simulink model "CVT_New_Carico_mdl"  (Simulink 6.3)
settings: Solver=ode15s  StartTime=0.0  StopTime=10.0  RelTol=1e-8  AbsTol=1e-8
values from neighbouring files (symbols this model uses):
  b_0 = kb*J_0    (= 0.00382059739779)    [CVT_New.m]    (also in CVT_New_th.m)
  b_mn = b_m+b_n*(Nm/Nn1)^2    (= 0.0609042388033)    [CVT_New.m]    (also in CVT_New_th.m)
  b_op = b_p+b_o*(Np/No)^2    (= 0.00942365042771)    [CVT_New.m]    (also in CVT_New_th.m)
  b_qt = b_q+b_t*(Nq/Nt1)^2    (= 0.0289383393218)    [CVT_New.m]    (also in CVT_New_th.m)
  b_r = kb*J_r    (= 218.026030555)    [architetture_epicicloidale_statico.m]    (also in architetture_HEV_startstop_1.m = 21.8026030555; architetture_HEV_startstop_2.m = 21.8026030555; CVT_New.m = 0.218026030555; CVT_New_th.m = 0.218026030555)
  Bs0 = diag([b_s,b_s0])    [CVT_New.m]    (also in CVT_New_th.m)
  C_pq = 1e-14*m^3/Pa    (= 1e-14)    [CVT_New.m]    (also in CVT_New_th.m)
  d_0s = d0    (= 10)    [CVT_New.m]    (also in CVT_New_th.m)
  d_m0 = d0    (= 10)    [CVT_New.m]    (also in CVT_New_th.m)
  d_pm = d0    (= 10)    [CVT_New.m]    (also in CVT_New_th.m)
  d_qr = d0    (= 10)    [CVT_New.m]    (also in CVT_New_th.m)
  d_sr = d0    (= 10)    [CVT_New.m]    (also in CVT_New_th.m; architetture_epicicloidale.m; architetture_epicicloidale_cont.m; architetture_epicicloidale_prova.m)
  Hp_max = Hq    (= 1.8724110952e-05)    [CVT_New.m]    (also in CVT_New_th.m)
  Hq = (400*lt/minuti)/(3400*rpm)    (= 1.8724110952e-05)    [CVT_New.m]    (also in CVT_New_th.m)
  J_0 = 1.3*0.5*pi*rho_acc*h0*r_0^4    (= 3.82059739779e-05)    [CVT_New.m]    (also in CVT_New_th.m)
  J_mn = J_m+J_n*(Nm/Nn1)^2    (= 0.000609042388033)    [CVT_New.m]    (also in CVT_New_th.m)
  J_op = J_p+J_o*(Np/No)^2    (= 9.42365042771e-05)    [CVT_New.m]    (also in CVT_New_th.m)
  J_qt = J_q+J_t*(Nq/Nt1)^2    (= 0.000289383393218)    [CVT_New.m]    (also in CVT_New_th.m)
  J_r = 0.5*pi*rho_acc*(hr*r_r^4 + h_ring*(r_re^4-r_r^4))    (= 2.18026030555)    [architetture_epicicloidale_statico.m]    (also in architetture_HEV_startstop_1.m; architetture_HEV_startstop_2.m; CVT_New.m = 0.00218026030555; CVT_New_th.m = 0.00218026030555)
  JJs0 = diag([J_s,J_s0])    [CVT_New.m]    (also in CVT_New_th.m)
  K_0s = K0    (= 1000000)    [CVT_New.m]    (also in CVT_New_th.m)
  K_m0 = K0    (= 1000000)    [CVT_New.m]    (also in CVT_New_th.m)
  K_pm = K0    (= 1000000)    [CVT_New.m]    (also in CVT_New_th.m)
  K_qr = K0    (= 1000000)    [CVT_New.m]    (also in CVT_New_th.m)
  K_sr = K0    (= 1000000)    [CVT_New.m]    (also in CVT_New_th.m; architetture_epicicloidale.m = 10000000; architetture_epicicloidale_cont.m = 10000000; architetture_epicicloidale_prova.m = 10000000)
  Mv = 4000*kg    (= 4000)    [CVT_New.m]    (also in CVT_New_th.m)
  Ppq_0 = 0    [CVT_New.m]    (also in CVT_New_th.m)
  r_0 = xd0*N0/(2*pi)    (= 0.0954929658551)    [CVT_New.m]    (also in CVT_New_th.m)
  r_mn = (Nm/Nn1)*r_n2    (= 0.148158783387)    [CVT_New.m]    (also in CVT_New_th.m)
  r_op = (Np/No)*r_o    (= 0.105042262441)    [CVT_New.m]    (also in CVT_New_th.m)
  R_p = 0.8*(30*bar)/(400*lt/minuti)    (= 360000000)    [CVT_New.m]    (also in CVT_New_th.m)
  R_q = 0.8*(30*bar)/(400*lt/minuti)    (= 360000000)    [CVT_New.m]    (also in CVT_New_th.m)
  r_qt = (Nq/Nt1)*r_t2    (= 0.111926639049)    [CVT_New.m]    (also in CVT_New_th.m)
  r_r1 = xdr*Nr1/(2*pi)    (= 0.248281711223)    [CVT_New.m]    (also in CVT_New_th.m)
  r_ri = xds*Nr2/(2*pi)    (= 0.248281711223)    [CVT_New.m]    (also in CVT_New_th.m; architetture_epicicloidale.m; architetture_epicicloidale_cont.m; architetture_epicicloidale_prova.m)
  Rr = 0.905*m    (= 0.905)    [CVT_New.m]    (also in CVT_New_th.m)
  Rs0 = [-r_s2;r_0]    [CVT_New.m]    (also in CVT_New_th.m)
  Rsr = [r_s1 r_ri]    [CVT_New.m]    (also in CVT_New_th.m)
  Tc = 0.05*ms    (= 5e-05)    [architetture_epicicloidale_statico.m]    (also in architetture_HEV_startstop_1.m; architetture_HEV_startstop_2.m; CVT_New.m; CVT_New_th.m)
  Tem = 440*N*m    (= 440)    [CVT_New.m]    (also in CVT_New_th.m)
  Tes = 0*N*m    (= 0)    [CVT_New.m]    (also in CVT_New_th.m)
  Tes0 = -0*(N0+Nr1)/N0*Tem*N*m    (= 0)    [CVT_New.m]    (also in CVT_New_th.m)
  Th_0 = 25*gradi    (= 0.436332312999)    [CVT_New.m]
  Th_max = 45*gradi    (= 0.785398163397)    [CVT_New.m]    (also in CVT_New_th.m)
  vetSLIPDry = [-0.7 -0.6 -0.5 -0.45 -0.4 -0.35 -0.3 -0.25 -0.2 -0.16 -0.14 -0.12 -0.1 -0.08 -0.06 -0.04 -0.02 0 0.02 0.04 0.06 0.08 0.1 0.12 0.14 0.16 0.2 0.25 0.3 0.35 0.4 0.45 0.5 0.6 0.7]'    [CVT_New.m]    (also in CVT_New_th.m)
  Vx_0 = ws0_0*Rr    [CVT_New.m]    (also in CVT_New_th.m)
  Vx_00 = 0.0000001    (= 1e-07)    [CVT_New.m]    (also in CVT_New_th.m)
  W0_0 = WW_0(2),    [CVT_New.m]    (also in CVT_New_th.m)
  Wm_0 = 1*rpm    (= 0.10471975512)    [CVT_New.m]    (also in CVT_New_th.m)
  Wp_0 = WW_0(6),    [CVT_New.m]    (also in CVT_New_th.m)
  Wq_0 = WW_0(7),    [CVT_New.m]    (also in CVT_New_th.m)
  Wr_0 = WW_0(5),    [CVT_New.m]    (also in CVT_New_th.m; architetture_epicicloidale.m = Sys1.C(3,:)*[Wc_0; Wsc_0]; Confronto_CVT_EMR.m = 0; epicicloidale.m = Sys1.C(3,:)*[Wc_0; Wsc_0])
  Ws0_0 = [ws_0;ws0_0]    [CVT_New.m]    (also in CVT_New_th.m)

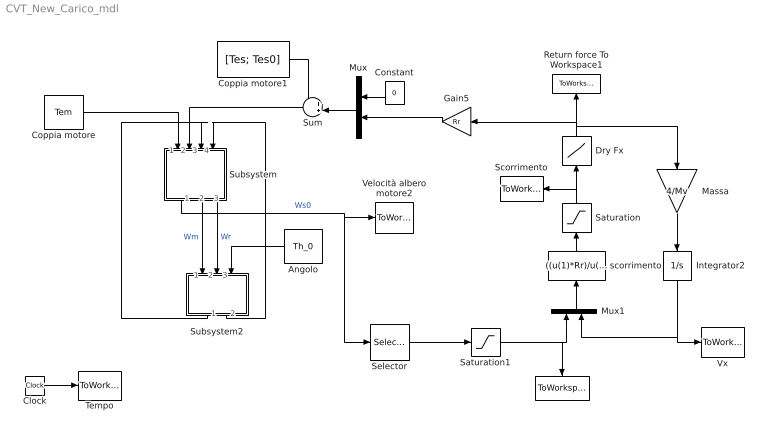
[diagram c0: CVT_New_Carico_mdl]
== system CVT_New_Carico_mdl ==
  " " : ToWorkspace  VariableName=Wr1  SampleTime=Tc  SaveFormat=Array
  Angolo : Constant  Orientation=left  Value=Th_0
  Clock : Clock
  Constant : Constant  Orientation=left  Value=0
  Coppia motore : Constant  Value=Tem
  Coppia motore1 : Constant  Value=[Tes; Tes0]
  Dry Fx : Lookup  Orientation=up  InputValues=vetSLIPDry  OutputValues=tabDryFX'
  Gain5 : Gain  Orientation=left  Gain=Rr
  Integrator2 : Integrator  Orientation=down  InitialCondition=Vx_0  LimitOutput=on  LowerSaturationLimit=Vx_00
  Massa : Gain  Orientation=down  Gain=4/Mv
  Mux : Mux  Orientation=left  Inputs=2
  Mux1 : Mux  Orientation=up  Inputs=2
  Return force To Workspace1 : ToWorkspace  VariableName=Fx  SampleTime=Tc  SaveFormat=Array
  Saturation : Saturate  Orientation=up  UpperLimit=0.7  LowerLimit=-0.7
  Saturation1 : Saturate  UpperLimit=inf  LowerLimit=0
  Scorrimento : ToWorkspace  VariableName=Slip  SampleTime=Tc  SaveFormat=Array
  Selector : Selector  Elements=[2]  InputPortWidth=2
  Subsystem : Subsystem  Orientation=down
  Subsystem2 : Subsystem  Orientation=down
  Sum : Sum  Orientation=left  Inputs=++|
  Tempo : ToWorkspace  VariableName=t  SampleTime=Tc  SaveFormat=Array
  Velocità albero motore2 : ToWorkspace  VariableName=Ws0  SampleTime=Tc  SaveFormat=Array
  Vx : ToWorkspace  VariableName=Vx  SampleTime=Tc  SaveFormat=Array
  scorrimento : Fcn  Orientation=up  Expr=((u(1)*Rr)/u(2))-1
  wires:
  Clock/1 -> Tempo/1
  Coppia motore/1 -> Subsystem/1(Tem)
  Sum/1 -> Subsystem/2(Ts0)
  Subsystem2/1(Tmn) -> Subsystem/3(Tmn)
  Subsystem2/2(Tr) -> Subsystem/4(Tr)
  Angolo/1 -> Subsystem2/3(Th)
  Subsystem/1(Ws0) -> Selector/1, Velocità albero motore2/1  "Ws0"
  Subsystem/2(Wm) -> Subsystem2/1(Wm)  "Wm"
  Subsystem/3(Wr) -> Subsystem2/2(Wr)  "Wr"
  Coppia motore1/1 -> Sum/1
  Mux/1 -> Sum/2
  Constant/1 -> Mux/1
  Massa/1 -> Integrator2/1
  Dry Fx/1 -> Gain5/1, Massa/1, Return force To Workspace1/1
  Saturation/1 -> Scorrimento/1, Dry Fx/1
  Integrator2/1 -> Vx/1, Mux1/2
  Saturation1/1 -> Mux1/1, " "/1
  scorrimento/1 -> Saturation/1
  Mux1/1 -> scorrimento/1
  Gain5/1 -> Mux/2
  Selector/1 -> Saturation1/1

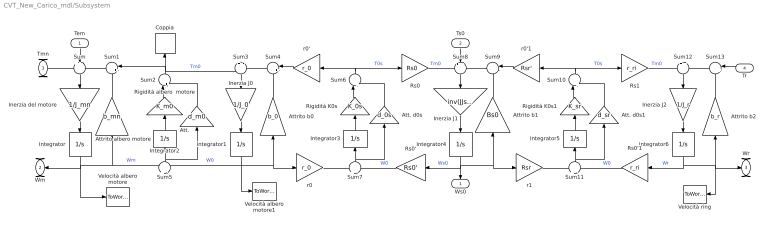
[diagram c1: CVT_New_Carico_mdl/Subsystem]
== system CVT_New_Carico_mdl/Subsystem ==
  Tem : Inport  Orientation=down
  Ts0 : Inport  Orientation=down  Port=2
  Tmn : Inport  Port=3
  Tr : Inport  Orientation=left  Port=4
  Att. : Gain  Orientation=up  Gain=d_m0
  Att. d0s : Gain  Orientation=up  Gain=d_0s
  Att. d0s1 : Gain  Orientation=up  Gain=d_sr
  Attrito albero motore : Gain  Orientation=up  Gain=b_mn
  Attrito b0 : Gain  Orientation=up  Gain=b_0
  Attrito b1 : Gain  Orientation=up  Gain=Bs0  Multiplication=Matrix(K*u)
  Attrito b2 : Gain  Orientation=up  Gain=b_r
  Coppia : ToWorkspace  VariableName=Tm0  SampleTime=Tc  SaveFormat=Array
  Inerzia J0 : Gain  Orientation=down  Gain=1/J_0
  Inerzia J1 : Gain  Orientation=down  Gain=inv(JJs0)  Multiplication=Matrix(K*u)
  Inerzia J2 : Gain  Orientation=down  Gain=1/J_r
  Inerzia del motore : Gain  Orientation=down  Gain=1/J_mn
  Integrator : Integrator  Orientation=down  InitialCondition=Wm_0  LowerSaturationLimit=0
  Integrator1 : Integrator  Orientation=down  InitialCondition=W0_0  LowerSaturationLimit=0
  Integrator2 : Integrator  Orientation=up
  Integrator3 : Integrator  Orientation=up
  Integrator4 : Integrator  Orientation=down  InitialCondition=Ws0_0  LowerSaturationLimit=0
  Integrator5 : Integrator  Orientation=up
  Integrator6 : Integrator  Orientation=down  InitialCondition=Wr_0  LowerSaturationLimit=0
  Rigidità K0s : Gain  Orientation=up  Gain=K_0s
  Rigidità K0s1 : Gain  Orientation=up  Gain=K_sr
  Rigidità albero  motore : Gain  Orientation=up  Gain=K_m0
  Rs0 : Gain  Gain=Rs0  Multiplication=Matrix(K*u)
  Rs0' : Gain  Orientation=left  Gain=Rs0'  Multiplication=Matrix(K*u)
  Rs0'1 : Gain  Orientation=left  Gain=r_ri
  Rs1 : Gain  Gain=r_ri
  Sum : Sum  Orientation=down  Inputs=++-
  Sum{1,4,9,13} (4 alike) : Sum  Orientation=left  Inputs=|++
  Sum10 : Sum  Orientation=up  Inputs=|++
  Sum11 : Sum  Orientation=up  Inputs=+|-
  Sum12 : Sum  Orientation=down  Inputs=+|-
  Sum2 : Sum  Orientation=up  Inputs=|++
  Sum3 : Sum  Orientation=down  Inputs=+|-
  Sum5 : Sum  Orientation=up  Inputs=+|-
  Sum6 : Sum  Orientation=up  Inputs=|++
  Sum7 : Sum  Orientation=up  Inputs=+|-
  Sum8 : Sum  Orientation=down  Inputs=+--
  Velocità albero motore : ToWorkspace  VariableName=Wm  SampleTime=Tc  SaveFormat=Array
  Velocità albero motore1 : ToWorkspace  VariableName=W0  SampleTime=Tc  SaveFormat=Array
  Velocità ring : ToWorkspace  VariableName=Wr  SampleTime=Tc  SaveFormat=Array
  r0 : Gain  Gain=r_0
  r0' : Gain  Orientation=left  Gain=r_0
  r0'1 : Gain  Orientation=left  Gain=Rsr'  Multiplication=Matrix(K*u)
  r1 : Gain  Gain=Rsr  Multiplication=Matrix(K*u)
  Ws0 : Outport  Orientation=down
  Wm : Outport  Orientation=left  Port=2
  Wr : Outport  Port=3
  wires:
  Sum/1 -> Inerzia del motore/1
  Inerzia del motore/1 -> Integrator/1
  Integrator/1 -> Attrito albero motore/1, Sum5/1, Wm/1, Velocità albero motore/1  "Wm"
  Attrito albero motore/1 -> Sum1/2
  Sum5/1 -> Integrator2/1, Att./1
  Sum2/1 -> Sum1/1, Sum3/1, Coppia/1  "Tm0"
  Sum1/1 -> Sum/3
  Integrator2/1 -> Rigidità albero  motore/1
  Rigidità albero  motore/1 -> Sum2/1
  Att./1 -> Sum2/2
  Sum3/1 -> Inerzia J0/1
  Inerzia J0/1 -> Integrator1/1
  Integrator1/1 -> Sum5/2, Attrito b0/1, r0/1, Velocità albero motore1/1  "W0"
  Attrito b0/1 -> Sum4/2
  r0'/1 -> Sum4/1
  Sum7/1 -> Att. d0s/1, Integrator3/1
  Sum6/1 -> r0'/1, Rs0/1  "T0s"
  Integrator3/1 -> Rigidità K0s/1
  Rigidità K0s/1 -> Sum6/1
  Att. d0s/1 -> Sum6/2
  Rs0'/1 -> Sum7/2  "W0"
  r0/1 -> Sum7/1
  Sum8/1 -> Inerzia J1/1
  Inerzia J1/1 -> Integrator4/1
  Integrator4/1 -> r1/1, Attrito b1/1, Rs0'/1, Ws0/1  "Ws0"
  Attrito b1/1 -> Sum9/2
  r0'1/1 -> Sum9/1
  Sum11/1 -> Integrator5/1, Att. d0s1/1
  Sum10/1 -> Rs1/1, r0'1/1  "T0s"
  Integrator5/1 -> Rigidità K0s1/1
  Rigidità K0s1/1 -> Sum10/1
  Att. d0s1/1 -> Sum10/2
  Rs0'1/1 -> Sum11/2  "W0"
  r1/1 -> Sum11/1
  Rs1/1 -> Sum12/1  "Tm0"
  Sum12/1 -> Inerzia J2/1
  Inerzia J2/1 -> Integrator6/1
  Integrator6/1 -> Attrito b2/1, Velocità ring/1, Wr/1, Rs0'1/1  "Wr"
  Attrito b2/1 -> Sum13/2
  Sum13/1 -> Sum12/2
  Sum9/1 -> Sum8/3
  Rs0/1 -> Sum8/1  "Tm0"
  Tem/1 -> Sum/2
  Ts0/1 -> Sum8/2
  Tmn/1 -> Sum/1
  Tr/1 -> Sum13/1
  Sum4/1 -> Sum3/2

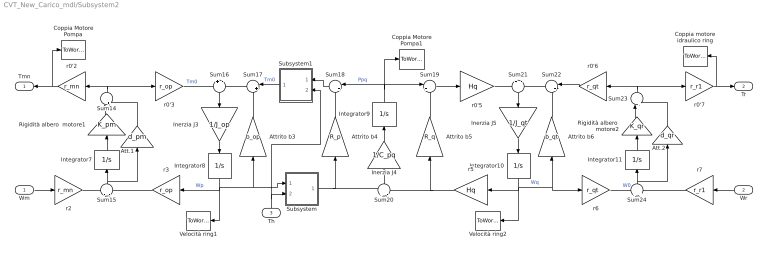
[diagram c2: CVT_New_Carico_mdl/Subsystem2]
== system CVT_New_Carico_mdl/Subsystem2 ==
  Wm : Inport
  Wr : Inport  Orientation=left  Port=2
  Th : Inport  Orientation=up  Port=3
  Att.1 : Gain  Orientation=up  Gain=d_pm
  Att.2 : Gain  Orientation=up  Gain=d_qr
  Attrito b3 : Gain  Orientation=up  Gain=b_op
  Attrito b4 : Gain  Orientation=up  Gain=R_p
  Attrito b5 : Gain  Orientation=up  Gain=R_q
  Attrito b6 : Gain  Orientation=up  Gain=b_qt
  Coppia motore idraulico ring : ToWorkspace  VariableName=Tqr  SampleTime=Tc  SaveFormat=Array
  Coppia Motore Pompa : ToWorkspace  VariableName=Tpm  SampleTime=Tc  SaveFormat=Array
  Coppia Motore Pompa1 : ToWorkspace  VariableName=Ppq  SampleTime=Tc  SaveFormat=Array
  Inerzia J3 : Gain  Orientation=down  Gain=1/J_op
  Inerzia J4 : Gain  Orientation=up  Gain=1/C_pq
  Inerzia J5 : Gain  Orientation=down  Gain=1/J_qt
  Integrator10 : Integrator  Orientation=down  InitialCondition=Wq_0  LowerSaturationLimit=0
  Integrator11 : Integrator  Orientation=up
  Integrator7 : Integrator  Orientation=up
  Integrator8 : Integrator  Orientation=down  InitialCondition=Wp_0  LowerSaturationLimit=0
  Integrator9 : Integrator  Orientation=up  InitialCondition=Ppq_0  LowerSaturationLimit=0
  Rigidità albero  motore1 : Gain  Orientation=up  Gain=K_pm
  Rigidità albero  motore2 : Gain  Orientation=up  Gain=K_qr
  Subsystem : Subsystem
  Subsystem1 : Subsystem  Orientation=left
  Sum14 : Sum  Orientation=up  Inputs=|++
  Sum15 : Sum  Orientation=up  Inputs=-|-
  Sum16 : Sum  Orientation=down  Inputs=+|-
  Sum17 : Sum  Orientation=left  Inputs=|++
  Sum18 : Sum  Orientation=left  Inputs=|++
  Sum19 : Sum  Inputs=|+-
  Sum20 : Sum  Orientation=up  Inputs=+|-
  Sum21 : Sum  Orientation=down  Inputs=+|-
  Sum22 : Sum  Orientation=left  Inputs=|++
  Sum23 : Sum  Orientation=up  Inputs=|++
  Sum24 : Sum  Orientation=up  Inputs=+|+
  Velocità ring1 : ToWorkspace  VariableName=Wp  SampleTime=Tc  SaveFormat=Array
  Velocità ring2 : ToWorkspace  VariableName=Wq  SampleTime=Tc  SaveFormat=Array
  r0'2 : Gain  Orientation=left  Gain=r_mn
  r0'3 : Gain  Gain=r_op
  r0'5 : Gain  Gain=Hq
  r0'6 : Gain  Orientation=left  Gain=r_qt
  r0'7 : Gain  Gain=r_r1
  r2 : Gain  Gain=r_mn
  r3 : Gain  Orientation=left  Gain=r_op
  r5 : Gain  Orientation=left  Gain=Hq
  r6 : Gain  Gain=r_qt
  r7 : Gain  Orientation=left  Gain=r_r1
  Tmn : Outport  Orientation=left
  Tr : Outport  Port=2
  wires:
  Sum15/1 -> Integrator7/1, Att.1/1
  Integrator7/1 -> Rigidità albero  motore1/1
  Rigidità albero  motore1/1 -> Sum14/1
  Att.1/1 -> Sum14/2
  r0'2/1 -> Coppia Motore Pompa/1, Tmn/1
  r2/1 -> Sum15/1
  Sum14/1 -> r0'2/1, r0'3/1
  r3/1 -> Sum15/2
  r0'3/1 -> Sum16/1  "Tm0"
  Sum16/1 -> Inerzia J3/1
  Inerzia J3/1 -> Integrator8/1
  Integrator8/1 -> Attrito b3/1, Subsystem/1(In1), r3/1, Velocità ring1/1  "Wp"
  Attrito b3/1 -> Sum17/2
  Sum17/1 -> Sum16/2
  Subsystem1/1(Out1) -> Sum17/1  "Tm0"
  Subsystem/1(Out1) -> Attrito b4/1, Sum20/1
  Attrito b4/1 -> Sum18/2
  Sum18/1 -> Subsystem1/1(In1)
  Attrito b5/1 -> Sum19/2
  Sum20/1 -> Inerzia J4/1
  Inerzia J4/1 -> Integrator9/1
  Integrator9/1 -> Sum18/1, Sum19/1, Coppia Motore Pompa1/1  "Ppq"
  Sum19/1 -> r0'5/1
  r5/1 -> Sum20/2, Attrito b5/1
  Sum21/1 -> Inerzia J5/1
  Inerzia J5/1 -> Integrator10/1
  Attrito b6/1 -> Sum22/2
  r0'5/1 -> Sum21/1
  Integrator10/1 -> r5/1, Attrito b6/1, r6/1, Velocità ring2/1  "Wq"
  r0'6/1 -> Sum22/1
  Sum22/1 -> Sum21/2
  Sum24/1 -> Integrator11/1, Att.2/1
  Integrator11/1 -> Rigidità albero  motore2/1
  Rigidità albero  motore2/1 -> Sum23/1
  Att.2/1 -> Sum23/2
  r6/1 -> Sum24/1  "W0"
  Sum23/1 -> r0'7/1, r0'6/1
  r7/1 -> Sum24/2
  r0'7/1 -> Coppia motore idraulico ring/1, Tr/1
  Th/1 -> Subsystem1/2(In2), Subsystem/2(In2)
  Wm/1 -> r2/1
  Wr/1 -> r7/1

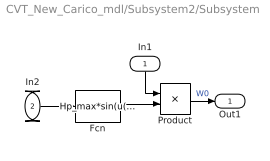
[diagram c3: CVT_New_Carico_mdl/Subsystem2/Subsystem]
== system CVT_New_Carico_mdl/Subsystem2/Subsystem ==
  In1 : Inport  Orientation=down
  In2 : Inport  Port=2
  Fcn : Fcn  Expr=Hp_max*sin(u(1))/sin(Th_max)
  Product : Product
  Out1 : Outport
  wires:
  In2/1 -> Fcn/1
  Fcn/1 -> Product/2
  In1/1 -> Product/1
  Product/1 -> Out1/1  "W0"

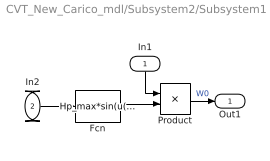
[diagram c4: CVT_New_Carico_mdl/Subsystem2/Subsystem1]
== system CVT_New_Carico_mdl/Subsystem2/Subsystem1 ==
  In1 : Inport  Orientation=down
  In2 : Inport  Port=2
  Fcn : Fcn  Expr=Hp_max*sin(u(1))/sin(Th_max)
  Product : Product
  Out1 : Outport
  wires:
  Product/1 -> Out1/1  "W0"
  In1/1 -> Product/1
  Fcn/1 -> Product/2
  In2/1 -> Fcn/1
